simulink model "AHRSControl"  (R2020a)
settings: Solver=FixedStepDiscrete  StartTime=0.0  StopTime=10.0  FixedStep=0.01  RelTol=1e-3  EnableMultiTasking=on
model workspace (MAT data in the model file):
  Ts : Simulink.Parameter (value not decoded)
symbols that are objects in the model workspace (value not decoded): Ts
undefined symbols (not defined in the file or in its folder): DiscIntNeverNeededParam
libraries: simulink x2

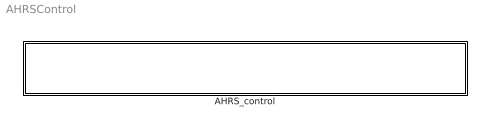
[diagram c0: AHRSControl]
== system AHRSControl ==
  AHRS_control : Subsystem  TreatAsAtomicUnit=on

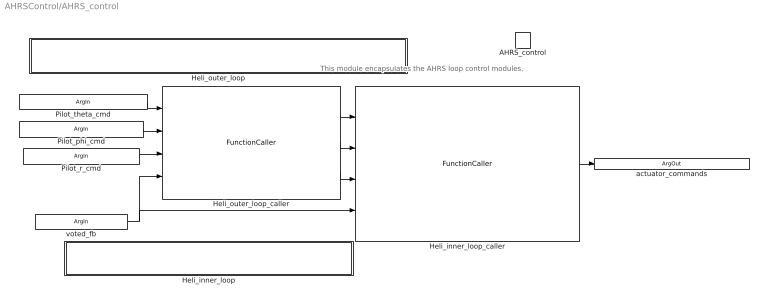
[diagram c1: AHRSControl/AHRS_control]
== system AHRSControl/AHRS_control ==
  note: This module encapsulates the AHRS loop control modules.
  AHRS_control : TriggerPort  TriggerType=function-call  IsSimulinkFunction=on  FunctionName=AHRS_control  FunctionVisibility=scoped  VariantControl=Variant  PortDimensions=1
  Heli_inner_loop : Subsystem  TreatAsAtomicUnit=on
  Heli_inner_loop_caller : FunctionCaller  FunctionPrototype=actuator_commands = Heli_inner_loop(theta_cmd,phi_cmd,r_cmd,voted_fb)
  Heli_outer_loop : Subsystem  TreatAsAtomicUnit=on
  Heli_outer_loop_caller : FunctionCaller  FunctionPrototype=[theta_cmd,phi_cmd,r_cmd] = Heli_outer_loop(Pilot_theta_cmd,Pilot_phi_cmd,Pilot_r_cmd,voted_fb)
  Pilot_theta_cmd : ArgIn  OutDataTypeStr=int16  ArgumentName=Pilot_theta_cmd
  Pilot_phi_cmd : ArgIn  Port=2  OutDataTypeStr=int16  ArgumentName=Pilot_phi_cmd
  Pilot_r_cmd : ArgIn  Port=3  OutDataTypeStr=int16  ArgumentName=Pilot_r_cmd
  voted_fb : ArgIn  Port=4  PortDimensions=5  ArgumentName=voted_fb
  actuator_commands : ArgOut  PortDimensions=3  ArgumentName=actuator_commands
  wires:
  Pilot_phi_cmd/1 -> Heli_outer_loop_caller/2
  Heli_outer_loop_caller/3 -> Heli_inner_loop_caller/3
  Heli_outer_loop_caller/1 -> Heli_inner_loop_caller/1
  Heli_inner_loop_caller/1 -> actuator_commands/1
  Heli_outer_loop_caller/2 -> Heli_inner_loop_caller/2
  voted_fb/1 -> Heli_outer_loop_caller/4, Heli_inner_loop_caller/4
  Pilot_r_cmd/1 -> Heli_outer_loop_caller/3
  Pilot_theta_cmd/1 -> Heli_outer_loop_caller/1

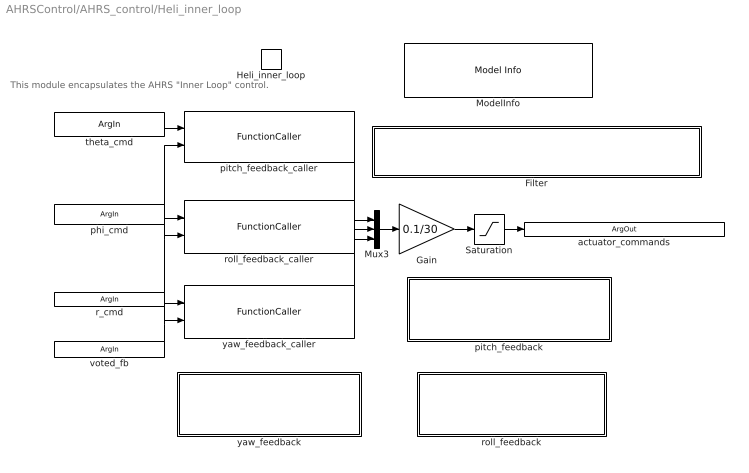
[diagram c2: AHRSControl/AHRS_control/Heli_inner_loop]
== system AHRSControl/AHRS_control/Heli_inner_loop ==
  note: This module encapsulates the AHRS "Inner Loop" control.
  Heli_inner_loop : TriggerPort  TriggerType=function-call  IsSimulinkFunction=on  FunctionName=Heli_inner_loop  FunctionVisibility=scoped  VariantControl=Variant  PortDimensions=1
  Filter : Subsystem  Tag=FilterWizardSubSystem  RequirementInfo={} %GIDa_ac7f675d_0c04_474f_b6aa_16ea1999b46b  TreatAsAtomicUnit=on  RTWFcnName=InnerLoopFilter
  Gain : Gain  Gain=0.1/30
  ModelInfo : simulink/Model-Wide Utilities/Model Info  Frame=on  DisplayStringWithTags=|  HorizontalTextAlignment=Center  LeftAlignmentValue=0.5
      | Model Name: %<ModelName>
      | Model Version: %<ModelVersion>
      | Last Modified: %<LastModificationDate>
      | 
      | Copyright 2016 The MathWorks, Inc.
  Mux3 : Mux  Inputs=3
  Saturation : Saturate  UpperLimit=0.1  LowerLimit=-0.1
  pitch_feedback : Subsystem  TreatAsAtomicUnit=on
  pitch_feedback_caller : FunctionCaller  FunctionPrototype=ds = pitch_feedback(theta_cmd,voted_fb)
  roll_feedback : Subsystem  TreatAsAtomicUnit=on
  roll_feedback_caller : FunctionCaller  FunctionPrototype=dc = roll_feedback(phi_cmd,voted_fb)
  yaw_feedback : Subsystem  TreatAsAtomicUnit=on
  yaw_feedback_caller : FunctionCaller  FunctionPrototype=dT = yaw_feedback(r_cmd,voted_fb)
  theta_cmd : ArgIn  ArgumentName=theta_cmd
  phi_cmd : ArgIn  Port=2  ArgumentName=phi_cmd
  r_cmd : ArgIn  Port=3  ArgumentName=r_cmd
  voted_fb : ArgIn  Port=4  PortDimensions=5  ArgumentName=voted_fb
  actuator_commands : ArgOut  PortDimensions=3  ArgumentName=actuator_commands
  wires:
  voted_fb/1 -> pitch_feedback_caller/2, roll_feedback_caller/2, yaw_feedback_caller/2
  Saturation/1 -> actuator_commands/1
  Gain/1 -> Saturation/1
  Mux3/1 -> Gain/1
  theta_cmd/1 -> pitch_feedback_caller/1
  phi_cmd/1 -> roll_feedback_caller/1
  r_cmd/1 -> yaw_feedback_caller/1
  roll_feedback_caller/1 -> Mux3/2
  yaw_feedback_caller/1 -> Mux3/3
  pitch_feedback_caller/1 -> Mux3/1

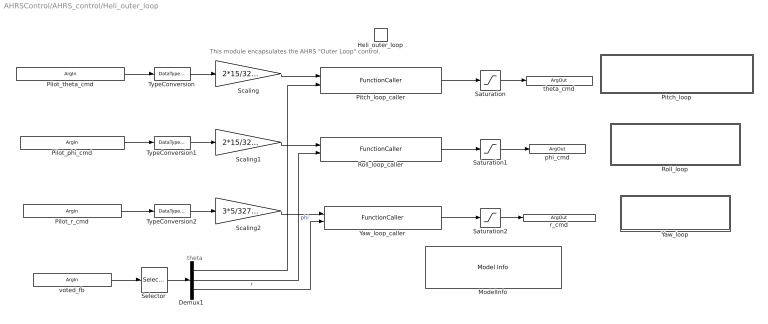
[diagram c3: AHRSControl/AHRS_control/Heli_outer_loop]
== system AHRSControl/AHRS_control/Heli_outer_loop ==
  note: theta
  note: This module encapsulates the AHRS "Outer Loop" control.
  Heli_outer_loop : TriggerPort  TriggerType=function-call  IsSimulinkFunction=on  FunctionName=Heli_outer_loop  FunctionVisibility=scoped  VariantControl=Variant  PortDimensions=1
  Demux1 : Demux  Outputs=3
  ModelInfo : simulink/Model-Wide Utilities/Model Info  Frame=on  DisplayStringWithTags=|  HorizontalTextAlignment=Center  LeftAlignmentValue=0.5
      | Model Name: %<ModelName>
      | Model Version: %<ModelVersion>
      | Last Modified: %<LastModificationDate>
      | 
      | Copyright 2016 The MathWorks, Inc.
  Pitch_loop : Subsystem  TreatAsAtomicUnit=on
  Pitch_loop_caller : FunctionCaller  FunctionPrototype=theta_cmd = Pitch_loop(Pilot_theta_cmd,theta)  InputArgumentSpecifications=double(1),double(1)  OutputArgumentSpecifications=double(1)
  Roll_loop : Subsystem  TreatAsAtomicUnit=on
  Roll_loop_caller : FunctionCaller  FunctionPrototype=phi_cmd = Roll_loop(Pilot_phi_cmd,phi)  InputArgumentSpecifications=double(1),double(1)  OutputArgumentSpecifications=double(1)
  Saturation : Saturate  UpperLimit=30  LowerLimit=-30
  Saturation1 : Saturate  UpperLimit=30  LowerLimit=-30
  Saturation2 : Saturate  UpperLimit=30  LowerLimit=-30
  Scaling : Gain  Gain=2*15/32767
  Scaling1 : Gain  Gain=2*15/32767
  Scaling2 : Gain  Gain=3*5/32767
  Selector : Selector  InputPortWidth=5  IndexOptions=Index vector (dialog)  Indices=[1 2 3]  OutputSizes=1
  TypeConversion : DataTypeConversion  OutDataTypeStr=double
  TypeConversion1 : DataTypeConversion  OutDataTypeStr=double
  TypeConversion2 : DataTypeConversion  OutDataTypeStr=double
  Yaw_loop : Subsystem  TreatAsAtomicUnit=on
  Yaw_loop_caller : FunctionCaller  FunctionPrototype=r_cmd = Yaw_loop(Pilot_r_cmd,r)  InputArgumentSpecifications=double(1), double(1)  OutputArgumentSpecifications=double(1)
  Pilot_theta_cmd : ArgIn  OutDataTypeStr=int16  ArgumentName=Pilot_theta_cmd
  Pilot_phi_cmd : ArgIn  Port=2  OutDataTypeStr=int16  ArgumentName=Pilot_phi_cmd
  Pilot_r_cmd : ArgIn  Port=3  OutDataTypeStr=int16  ArgumentName=Pilot_r_cmd
  voted_fb : ArgIn  Port=4  PortDimensions=5  ArgumentName=voted_fb
  theta_cmd : ArgOut  ArgumentName=theta_cmd
  phi_cmd : ArgOut  Port=2  ArgumentName=phi_cmd
  r_cmd : ArgOut  Port=3  ArgumentName=r_cmd
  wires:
  Selector/1 -> Demux1/1
  TypeConversion2/1 -> Scaling2/1
  Pilot_r_cmd/1 -> TypeConversion2/1
  Pilot_phi_cmd/1 -> TypeConversion1/1
  Saturation1/1 -> phi_cmd/1
  TypeConversion1/1 -> Scaling1/1
  Saturation2/1 -> r_cmd/1
  voted_fb/1 -> Selector/1
  Roll_loop_caller/1 -> Saturation1/1
  Yaw_loop_caller/1 -> Saturation2/1
  TypeConversion/1 -> Scaling/1
  Saturation/1 -> theta_cmd/1
  Pilot_theta_cmd/1 -> TypeConversion/1
  Scaling/1 -> Pitch_loop_caller/1
  Demux1/1 -> Pitch_loop_caller/2
  Scaling1/1 -> Roll_loop_caller/1
  Demux1/2 -> Roll_loop_caller/2  "phi"
  Pitch_loop_caller/1 -> Saturation/1
  Scaling2/1 -> Yaw_loop_caller/1
  Demux1/3 -> Yaw_loop_caller/2  "r"

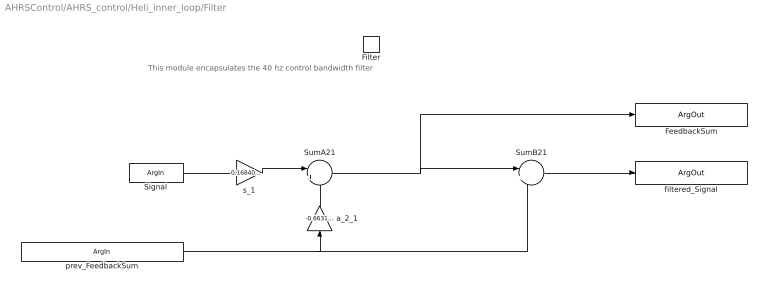
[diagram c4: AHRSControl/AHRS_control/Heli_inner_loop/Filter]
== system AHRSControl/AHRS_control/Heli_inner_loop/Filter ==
  note: This module encapsulates the 40 hz control bandwidth filter
  Filter : TriggerPort  TriggerType=function-call  IsSimulinkFunction=on  FunctionName=Filter  FunctionVisibility=scoped  VariantControl=Variant  PortDimensions=1
  SumA21 : Sum  Inputs=|+-  RndMeth=Zero  SaturateOnIntegerOverflow=on
  SumB21 : Sum  Inputs=|++  RndMeth=Zero  SaturateOnIntegerOverflow=on
  a_2_1 : Gain  Gain=-0.66319151740124993  ParamDataTypeStr=double  RndMeth=Zero  SaturateOnIntegerOverflow=on
  s_1 : Gain  Gain=0.16840424129937498  ParamDataTypeStr=double  RndMeth=Zero  SaturateOnIntegerOverflow=on
  Signal : ArgIn  ArgumentName=Signal
  prev_FeedbackSum : ArgIn  Port=2  ArgumentName=prev_FeedbackSum
  filtered_Signal : ArgOut  ArgumentName=filtered_Signal
  FeedbackSum : ArgOut  Port=2  ArgumentName=FeedbackSum
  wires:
  a_2_1/1 -> SumA21/2
  SumB21/1 -> filtered_Signal/1
  SumA21/1 -> FeedbackSum/1, SumB21/1
  s_1/1 -> SumA21/1
  Signal/1 -> s_1/1
  prev_FeedbackSum/1 -> SumB21/2, a_2_1/1

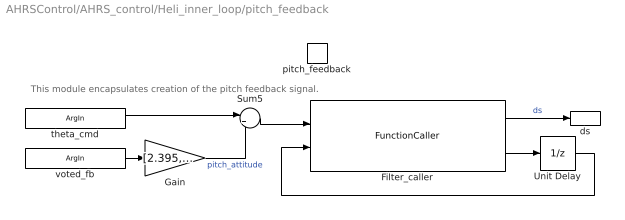
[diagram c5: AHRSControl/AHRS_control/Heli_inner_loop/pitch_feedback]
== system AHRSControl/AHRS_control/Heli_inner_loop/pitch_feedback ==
  note: This module encapsulates creation of the pitch feedback signal.
  pitch_feedback : TriggerPort  TriggerType=function-call  IsSimulinkFunction=on  FunctionName=pitch_feedback  FunctionVisibility=scoped  VariantControl=Variant  PortDimensions=1
  Filter_caller : FunctionCaller  FunctionPrototype=[filtered_Signal,FeedbackSum] = Filter(Signal,prev_FeedbackSum)  InputArgumentSpecifications=double(1), double(1)  OutputArgumentSpecifications=double(1), double(1)
  Gain : Gain  Gain=[2.395,-0.3609,-0.002145,0.808700,-0.0205;;]  Multiplication=Matrix(K*u) (u vector)
  Sum5 : Sum  Inputs=|+-
  Unit Delay : UnitDelay  SampleTime=-1  HasFrameUpgradeWarning=on
  theta_cmd : ArgIn  ArgumentName=theta_cmd
  voted_fb : ArgIn  Port=2  PortDimensions=5  ArgumentName=voted_fb
  ds : ArgOut  ArgumentName=ds
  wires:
  voted_fb/1 -> Gain/1
  theta_cmd/1 -> Sum5/1
  Sum5/1 -> Filter_caller/1
  Filter_caller/1 -> ds/1  "ds"
  Gain/1 -> Sum5/2  "pitch_attitude"
  Filter_caller/2 -> Unit Delay/1
  Unit Delay/1 -> Filter_caller/2

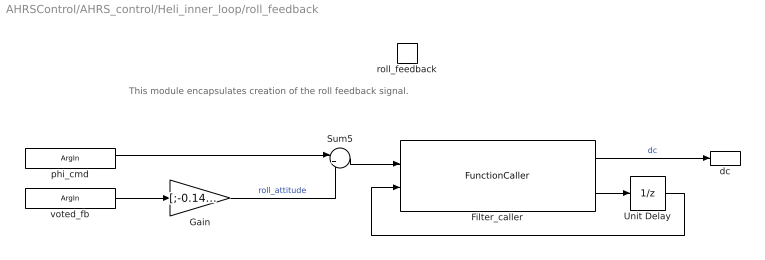
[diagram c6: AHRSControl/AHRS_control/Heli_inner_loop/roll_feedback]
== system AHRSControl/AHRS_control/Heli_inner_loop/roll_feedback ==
  note: This module encapsulates creation of the roll feedback signal.
  roll_feedback : TriggerPort  TriggerType=function-call  IsSimulinkFunction=on  FunctionName=roll_feedback  FunctionVisibility=scoped  VariantControl=Variant  PortDimensions=1
  Filter_caller : FunctionCaller  FunctionPrototype=[filtered_Signal,FeedbackSum] = Filter(Signal,prev_FeedbackSum)  InputArgumentSpecifications=double(1), double(1)  OutputArgumentSpecifications=double(1), double(1)
  Gain : Gain  Gain=[;-0.1427,-1.115,0.04573,-0.04318,-0.1007;]  Multiplication=Matrix(K*u) (u vector)
  Sum5 : Sum  Inputs=|+-
  Unit Delay : UnitDelay  SampleTime=-1  HasFrameUpgradeWarning=on
  phi_cmd : ArgIn  ArgumentName=phi_cmd
  voted_fb : ArgIn  Port=2  PortDimensions=5  ArgumentName=voted_fb
  dc : ArgOut  ArgumentName=dc
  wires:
  Unit Delay/1 -> Filter_caller/2
  Filter_caller/2 -> Unit Delay/1
  Gain/1 -> Sum5/2  "roll_attitude"
  Filter_caller/1 -> dc/1  "dc"
  Sum5/1 -> Filter_caller/1
  phi_cmd/1 -> Sum5/1
  voted_fb/1 -> Gain/1

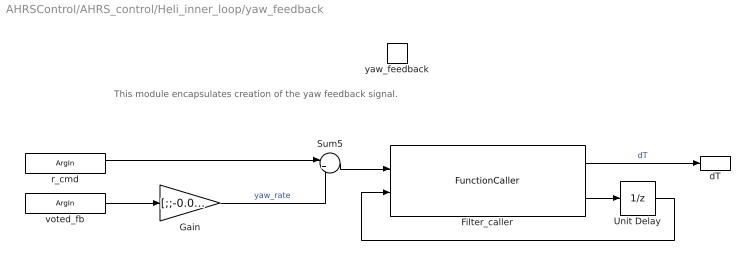
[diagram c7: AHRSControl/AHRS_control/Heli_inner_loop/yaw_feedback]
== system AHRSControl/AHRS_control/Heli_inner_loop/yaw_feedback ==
  note: This module encapsulates creation of the yaw feedback signal.
  yaw_feedback : TriggerPort  TriggerType=function-call  IsSimulinkFunction=on  FunctionName=yaw_feedback  FunctionVisibility=scoped  VariantControl=Variant  PortDimensions=1
  Filter_caller : FunctionCaller  FunctionPrototype=[filtered_Signal,FeedbackSum] = Filter(Signal,prev_FeedbackSum)  InputArgumentSpecifications=double(1), double(1)  OutputArgumentSpecifications=double(1), double(1)
  Gain : Gain  Gain=[;;-0.02792,-0.02229,-2.25,-0.06152,0.03151]  Multiplication=Matrix(K*u) (u vector)
  Sum5 : Sum  Inputs=|+-
  Unit Delay : UnitDelay  SampleTime=-1  HasFrameUpgradeWarning=on
  r_cmd : ArgIn  ArgumentName=r_cmd
  voted_fb : ArgIn  Port=2  PortDimensions=5  ArgumentName=voted_fb
  dT : ArgOut  ArgumentName=dT
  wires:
  voted_fb/1 -> Gain/1
  r_cmd/1 -> Sum5/1
  Sum5/1 -> Filter_caller/1
  Filter_caller/1 -> dT/1  "dT"
  Gain/1 -> Sum5/2  "yaw_rate"
  Filter_caller/2 -> Unit Delay/1
  Unit Delay/1 -> Filter_caller/2

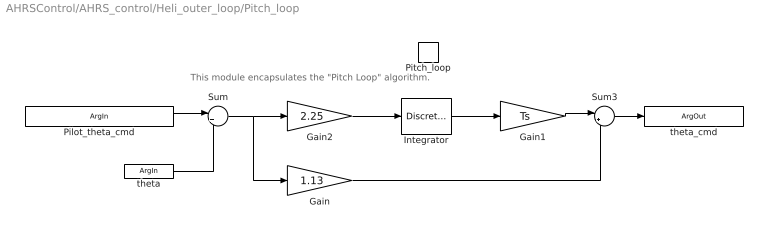
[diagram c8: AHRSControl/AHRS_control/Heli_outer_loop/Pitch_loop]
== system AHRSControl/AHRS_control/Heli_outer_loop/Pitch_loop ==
  note: This module encapsulates the "Pitch Loop" algorithm.
  Pitch_loop : TriggerPort  TriggerType=function-call  IsSimulinkFunction=on  FunctionName=Pitch_loop  FunctionVisibility=scoped  VariantControl=Variant  PortDimensions=1
  Gain : Gain  Gain=1.13
  Gain1 : Gain  Gain=Ts
  Gain2 : Gain  Gain=2.25
  Integrator : DiscreteIntegrator  IntegratorMethod=Accumulation: Forward Euler  SampleTime=-1  LimitOutput=on  UpperSaturationLimit=10  LowerSaturationLimit=-10  ICPrevOutput=DiscIntNeverNeededParam  ICPrevScaledInput=DiscIntNeverNeededParam
  Sum : Sum  Inputs=|+-  InputSameDT=on
  Sum3 : Sum  Inputs=|++
  Pilot_theta_cmd : ArgIn  ArgumentName=Pilot_theta_cmd
  theta : ArgIn  Port=2  ArgumentName=theta
  theta_cmd : ArgOut  ArgumentName=theta_cmd
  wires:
  Gain2/1 -> Integrator/1
  Sum3/1 -> theta_cmd/1
  Integrator/1 -> Gain1/1
  Gain/1 -> Sum3/2
  Gain1/1 -> Sum3/1
  Pilot_theta_cmd/1 -> Sum/1
  Sum/1 -> Gain/1, Gain2/1
  theta/1 -> Sum/2

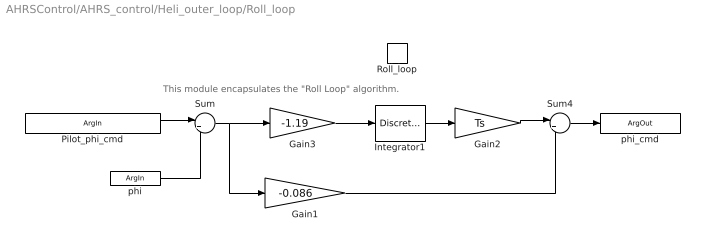
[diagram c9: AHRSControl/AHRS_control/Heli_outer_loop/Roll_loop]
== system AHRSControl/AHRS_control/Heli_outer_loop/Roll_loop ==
  note: This module encapsulates the "Roll Loop" algorithm.
  Roll_loop : TriggerPort  TriggerType=function-call  IsSimulinkFunction=on  FunctionName=Roll_loop  FunctionVisibility=scoped  VariantControl=Variant  PortDimensions=1
  Gain1 : Gain  Gain=-0.086
  Gain2 : Gain  Gain=Ts
  Gain3 : Gain  Gain=-1.19
  Integrator1 : DiscreteIntegrator  IntegratorMethod=Accumulation: Forward Euler  SampleTime=-1  LimitOutput=on  UpperSaturationLimit=10  LowerSaturationLimit=-10  ICPrevOutput=DiscIntNeverNeededParam  ICPrevScaledInput=DiscIntNeverNeededParam
  Sum : Sum  Inputs=|+-  InputSameDT=on
  Sum4 : Sum  Inputs=|++
  Pilot_phi_cmd : ArgIn  ArgumentName=Pilot_phi_cmd
  phi : ArgIn  Port=2  ArgumentName=phi
  phi_cmd : ArgOut  ArgumentName=phi_cmd
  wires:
  Sum4/1 -> phi_cmd/1
  Gain3/1 -> Integrator1/1
  Gain1/1 -> Sum4/2
  Integrator1/1 -> Gain2/1
  Gain2/1 -> Sum4/1
  phi/1 -> Sum/2
  Pilot_phi_cmd/1 -> Sum/1
  Sum/1 -> Gain1/1, Gain3/1

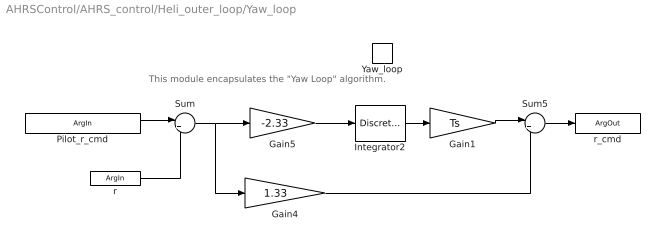
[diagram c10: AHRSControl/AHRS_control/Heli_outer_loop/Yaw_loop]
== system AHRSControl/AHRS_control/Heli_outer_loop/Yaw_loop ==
  note: This module encapsulates the "Yaw Loop" algorithm.
  Yaw_loop : TriggerPort  TriggerType=function-call  IsSimulinkFunction=on  FunctionName=Yaw_loop  FunctionVisibility=scoped  VariantControl=Variant  PortDimensions=1
  Gain1 : Gain  Gain=Ts
  Gain4 : Gain  Gain=1.33
  Gain5 : Gain  Gain=-2.33
  Integrator2 : DiscreteIntegrator  IntegratorMethod=Accumulation: Forward Euler  SampleTime=-1  LimitOutput=on  UpperSaturationLimit=10  LowerSaturationLimit=-10  ICPrevOutput=DiscIntNeverNeededParam  ICPrevScaledInput=DiscIntNeverNeededParam
  Sum : Sum  Inputs=|+-  InputSameDT=on
  Sum5 : Sum  Inputs=|++
  Pilot_r_cmd : ArgIn  ArgumentName=Pilot_r_cmd
  r : ArgIn  Port=2  ArgumentName=r
  r_cmd : ArgOut  ArgumentName=r_cmd
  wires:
  Integrator2/1 -> Gain1/1
  Gain4/1 -> Sum5/2
  Gain5/1 -> Integrator2/1
  Sum5/1 -> r_cmd/1
  Gain1/1 -> Sum5/1
  r/1 -> Sum/2
  Pilot_r_cmd/1 -> Sum/1
  Sum/1 -> Gain4/1, Gain5/1
